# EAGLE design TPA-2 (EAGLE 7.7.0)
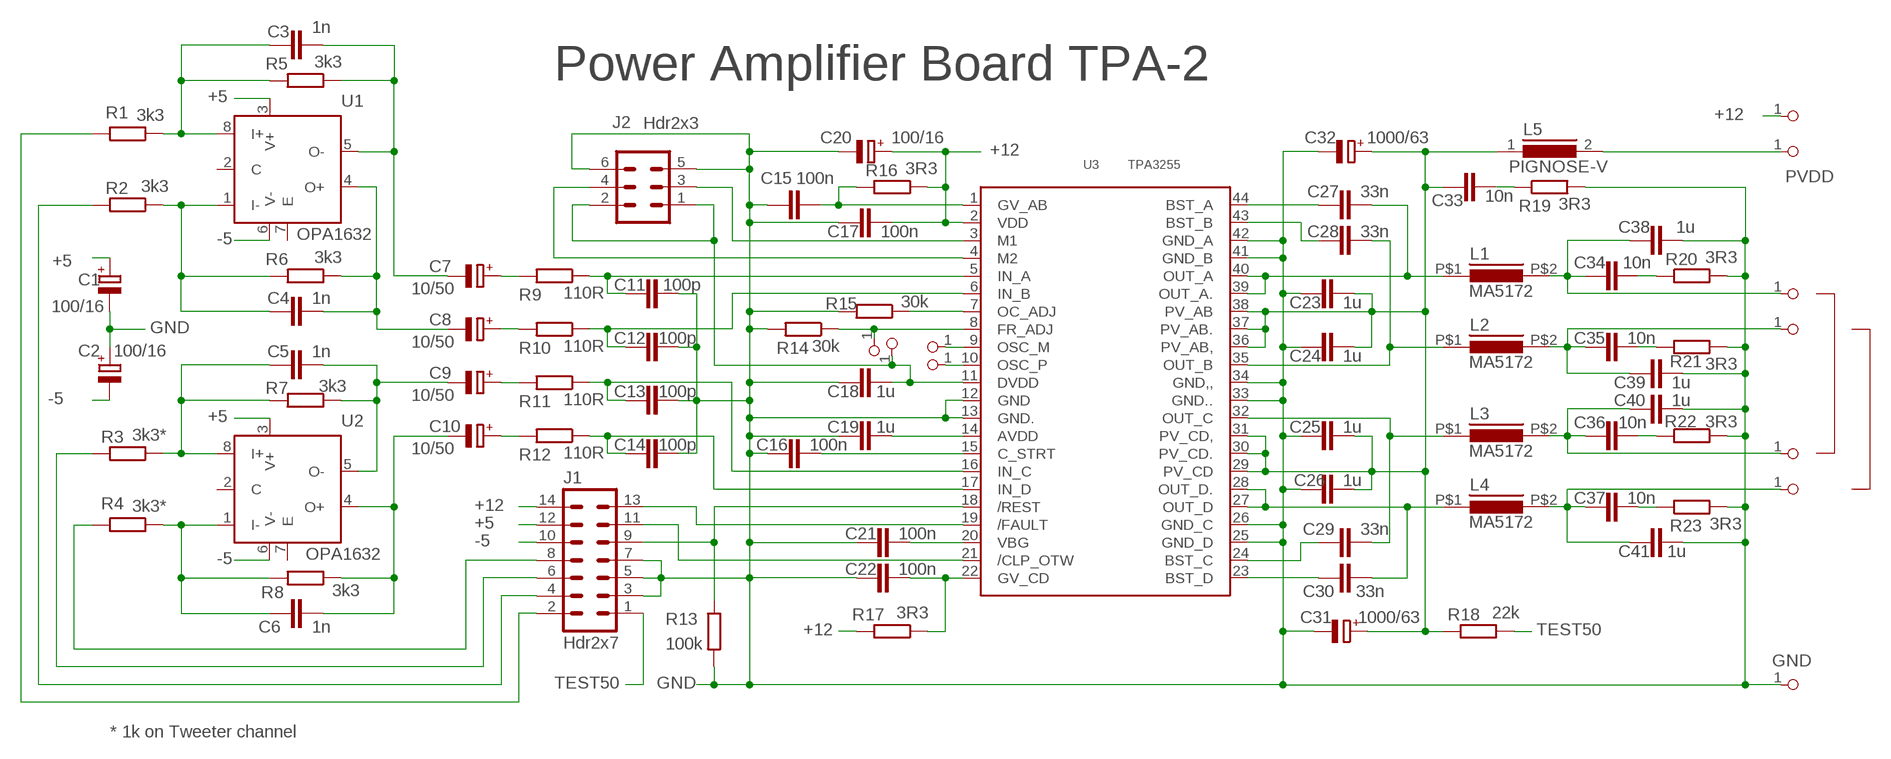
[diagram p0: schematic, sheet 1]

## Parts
12  PINHDR-1X1  [HDR1X1]
50  PINHDR-1X1  [HDR1X1]
A  PINHDR-1X1  [HDR1X1]
B  PINHDR-1X1  [HDR1X1]
C  PINHDR-1X1  [HDR1X1]
C1  100/16  CPOL-EUE2.5-6  [E2,5-6]
C2  100/16  CPOL-EUE2.5-6  [E2,5-6]
C3  1n  C-EUC0805  [C0805]
C4  1n  C-EUC0805  [C0805]
C5  1n  C-EUC0805  [C0805]
C6  1n  C-EUC0805  [C0805]
C7  10/50  CPOL-EUE2.5-6  [E2,5-6]
C8  10/50  CPOL-EUE2.5-6  [E2,5-6]
C9  10/50  CPOL-EUE2.5-6  [E2,5-6]
C10  10/50  CPOL-EUE2.5-6  [E2,5-6]
C11  100p  C-EUC0805  [C0805]
C12  100p  C-EUC0805  [C0805]
C13  100p  C-EUC0805  [C0805]
C14  100p  C-EUC0805  [C0805]
C15  100n  C-EUC1206  [C1206]
C16  100n  C-EUC1206  [C1206]
C17  100n  C-EUC1206  [C1206]
C18  1u  C-EUC1206  [C1206]
C19  1u  C-EUC1206  [C1206]
C20  100/16  CPOL-EUE2.5-6  [E2,5-6]
C21  100n  C-EUC1206  [C1206]
C22  100n  C-EUC1206  [C1206]
C23  1u  C-EUC1206  [C1206]
C24  1u  C-EUC1206  [C1206]
C25  1u  C-EUC1206  [C1206]
C26  1u  C-EUC1206  [C1206]
C27  33n  C-EUC1206  [C1206]
C28  33n  C-EUC1206  [C1206]
C29  33n  C-EUC1206  [C1206]
C30  33n  C-EUC1206  [C1206]
C31  1000/63  CPOL-EUE7.5-16  [E7,5-16]
C32  1000/63  CPOL-EUE7.5-16  [E7,5-16]
C33  10n  C-EUC1206  [C1206]
C34  10n  C-EUC1206  [C1206]
C35  10n  C-EUC1206  [C1206]
C36  10n  C-EUC1206  [C1206]
C37  10n  C-EUC1206  [C1206]
C38  1u  C-EU075-052X106  [C075-052X106]
C39  1u  C-EU075-052X106  [C075-052X106]
C40  1u  C-EU075-052X106  [C075-052X106]
C41  1u  C-EU075-052X106  [C075-052X106]
D  PINHDR-1X1  [HDR1X1]
DVDD  PINHDR-1X1  [HDR1X1]
FA  PINHDR-1X1  [HDR1X1]
G  PINHDR-1X1  [HDR1X1]
J1  Hdr2x7  PINHD-7X2  [MA07-2]
J2  Hdr2x3  PINHD-3X2  [MA03-2]
L1  MA5172  [L12X29]
L2  MA5172  [L12X29]
L3  MA5172  [L12X29]
L4  MA5172  [L12X29]
L5  PIGNOSE-V  INDUCTOR-PIGNOSE-V  [PIGNOSE]
OM  PINHDR-1X1  [HDR1X1]
OP  PINHDR-1X1  [HDR1X1]
R1  3k3  R-EU_0204/2V  [0204V]
R2  3k3  R-EU_0204/2V  [0204V]
R3  3k3*  R-EU_0204/2V  [0204V]
R4  3k3*  R-EU_0204/2V  [0204V]
R5  3k3  R-EU_0204/2V  [0204V]
R6  3k3  R-EU_0204/2V  [0204V]
R7  3k3  R-EU_0204/2V  [0204V]
R8  3k3  R-EU_0204/2V  [0204V]
R9  110R  R-EU_0204/2V  [0204V]
R10  110R  R-EU_0204/2V  [0204V]
R11  110R  R-EU_0204/2V  [0204V]
R12  110R  R-EU_0204/2V  [0204V]
R13  100k  R-EU_0204/2V  [0204V]
R14  30k  R-EU_0204/2V  [0204V]
R15  30k  R-EU_0204/2V  [0204V]
R16  3R3  R-EU_0204/2V  [0204V]
R17  3R3  R-EU_0204/2V  [0204V]
R18  22k  R-EU_0207/10  [0207/10]
R19  3R3  R-EU_0207/10  [0207/10]
R20  3R3  R-EU_0207/10  [0207/10]
R21  3R3  R-EU_0207/10  [0207/10]
R22  3R3  R-EU_0207/10  [0207/10]
R23  3R3  R-EU_0207/10  [0207/10]
U1  OPA1632  [SO08]
U2  OPA1632  [SO08]
U3  TPA3255  [HTSSOP-44]

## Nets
+5: C1.+ J1.12 U1.3(V+) U2.3(V+)
+12: 12.1 C17.2 C20.+ J1.14 R16.1 R17.2 U3.2(VDD)
-5: C2.- J1.10 U1.6(V-) U2.6(V-)
AVDD: C19.2 U3.14(AVDD)
BST_A: C27.1 U3.44(BST_A)
BST_B: C28.1 U3.43(BST_B)
BST_C: C29.1 U3.24(BST_C)
BST_D: C30.1 U3.23(BST_D)
CPLOTW: J1.11 U3.21(/CLP_OTW)
DVDD: C18.2 DVDD.1 J2.1 J2.2 U3.11(DVDD)
FLT: J1.13 U3.19(/FAULT)
FRADJ: FA.1 R14.1 U3.8(FR_ADJ)
GND: C1.- C2.+ C11.2 C12.2 C13.2 C14.2 C15.1 C16.1 C17.1 C18.1 C19.1 C20.- C21.1 C22.1 C23.1 C24.1 C25.1 C26.1 C31.- C32.- C38.1 C39.1 C40.1 C41.1 G.1 J1.3 J1.5 J1.7 J2.5 J2.6 R13.2 R14.2 R15.2 R19.2 R20.2 R21.2 R22.2 R23.2 U3.12(GND) U3.13(GND.) U3.25(GND_D) U3.26(GND_C) U3.33(GND..) U3.34(GND,,) U3.41(GND_B) U3.42(GND_A)
GVAB: C15.2 R16.2 U3.1(GV_AB)
GVCD: C22.2 R17.1 U3.22(GV_CD)
INA: C11.1 R9.1 U3.5(IN_A)
INB: C12.1 R10.1 U3.6(IN_B)
INC: C13.1 R11.1 U3.16(IN_C)
IND: C14.1 R12.1 U3.17(IN_D)
M1: J2.3 U3.3(M1)
M2: J2.4 U3.4(M2)
N$2: C37.1 R23.1
N$3: C37.2 C41.2 D.1 L4.P$2
N$4: A.1 C34.2 C38.2 L1.P$2
N$5: C36.2 C40.2 C.1 L3.P$2
N$9: B.1 C35.2 C39.2 L2.P$2
N$18: C7.+ R9.2
N$20: C34.1 R20.1
N$23: C35.1 R21.1
N$26: C3.1 R1.1 R5.2 U1.8(I+)
N$27: C36.1 R22.1
N$28: C33.1 R19.1
N$30: C8.+ R10.2
N$35: J1.8 R4.2
N$36: J1.6 R3.2
N$37: J1.4 R2.2
N$40: J1.2 R1.2
N$41: 50.1 L5.2
N$42: C9.+ R11.2
N$43: C10.+ R12.2
N$45: C4.1 R2.1 R6.2 U1.1(I-)
N$50: C4.2 C8.- R6.1 U1.4(O+)
N$51: C3.2 C7.- R5.1 U1.5(O-)
N$52: C5.2 C9.- R7.1 U2.5(O-)
N$53: C5.1 R3.1 R7.2 U2.8(I+)
N$55: C6.1 R4.1 R8.2 U2.1(I-)
N$56: C6.2 C10.- R8.1 U2.4(O+)
OM: OM.1 U3.9(OSC_M)
OP: OP.1 U3.10(OSC_P)
OSCADJ: R15.1 U3.7(OC_ADJ)
OUT_A: C27.2 L1.P$1 U3.39(OUT_A.) U3.40(OUT_A)
OUT_B: C28.2 L2.P$1 U3.35(OUT_B)
OUT_C: C29.2 L3.P$1 U3.32(OUT_C)
OUT_D: C30.2 L4.P$1 U3.27(OUT_D) U3.28(OUT_D.)
PVDD: C23.2 C24.2 C25.2 C26.2 C31.+ C32.+ C33.2 L5.1 R18.1 U3.29(PV_CD) U3.30(PV_CD.) U3.31(PV_CD,) U3.36(PV_AB,) U3.37(PV_AB.) U3.38(PV_AB)
RST: J1.9 R13.1 U3.18(/REST)
STRT: C16.2 U3.15(C_STRT)
TEST50: J1.1 R18.2
VBG: C21.2 U3.20(VBG)
Unconnected: U1.2(C) U1.7(E) U2.2(C) U2.7(E)

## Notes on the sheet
- Power Amplifier Board TPA-2
- * 1k on Tweeter channel

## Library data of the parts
12 50 A B C D DVDD FA G OM OP = Header:PINHDR-1X1
C1 C2 C7-C10 C20 C31 C32 = Passive:CPOL-EU: POLARIZED CAPACITOR, European symbol
C3-C6 C11-C19 C21-C30 C33-C41 = Passive:C-EU: CAPACITOR, European symbol
J1 = Header:PINHD-7X2: PIN HEADER
J2 = Header:PINHD-3X2: PIN HEADER
L1-L4 = Passive:MA5172
L5 = Passive:INDUCTOR: INDUCTOR
R1-R23 = AJANLIB:R-EU_: RESISTOR, European symbol
U1 U2 = IC_Lin:OPA1632
U3 = MotorDrive:TPA3255: 4-2-1 Channel Class D Audio Power stage

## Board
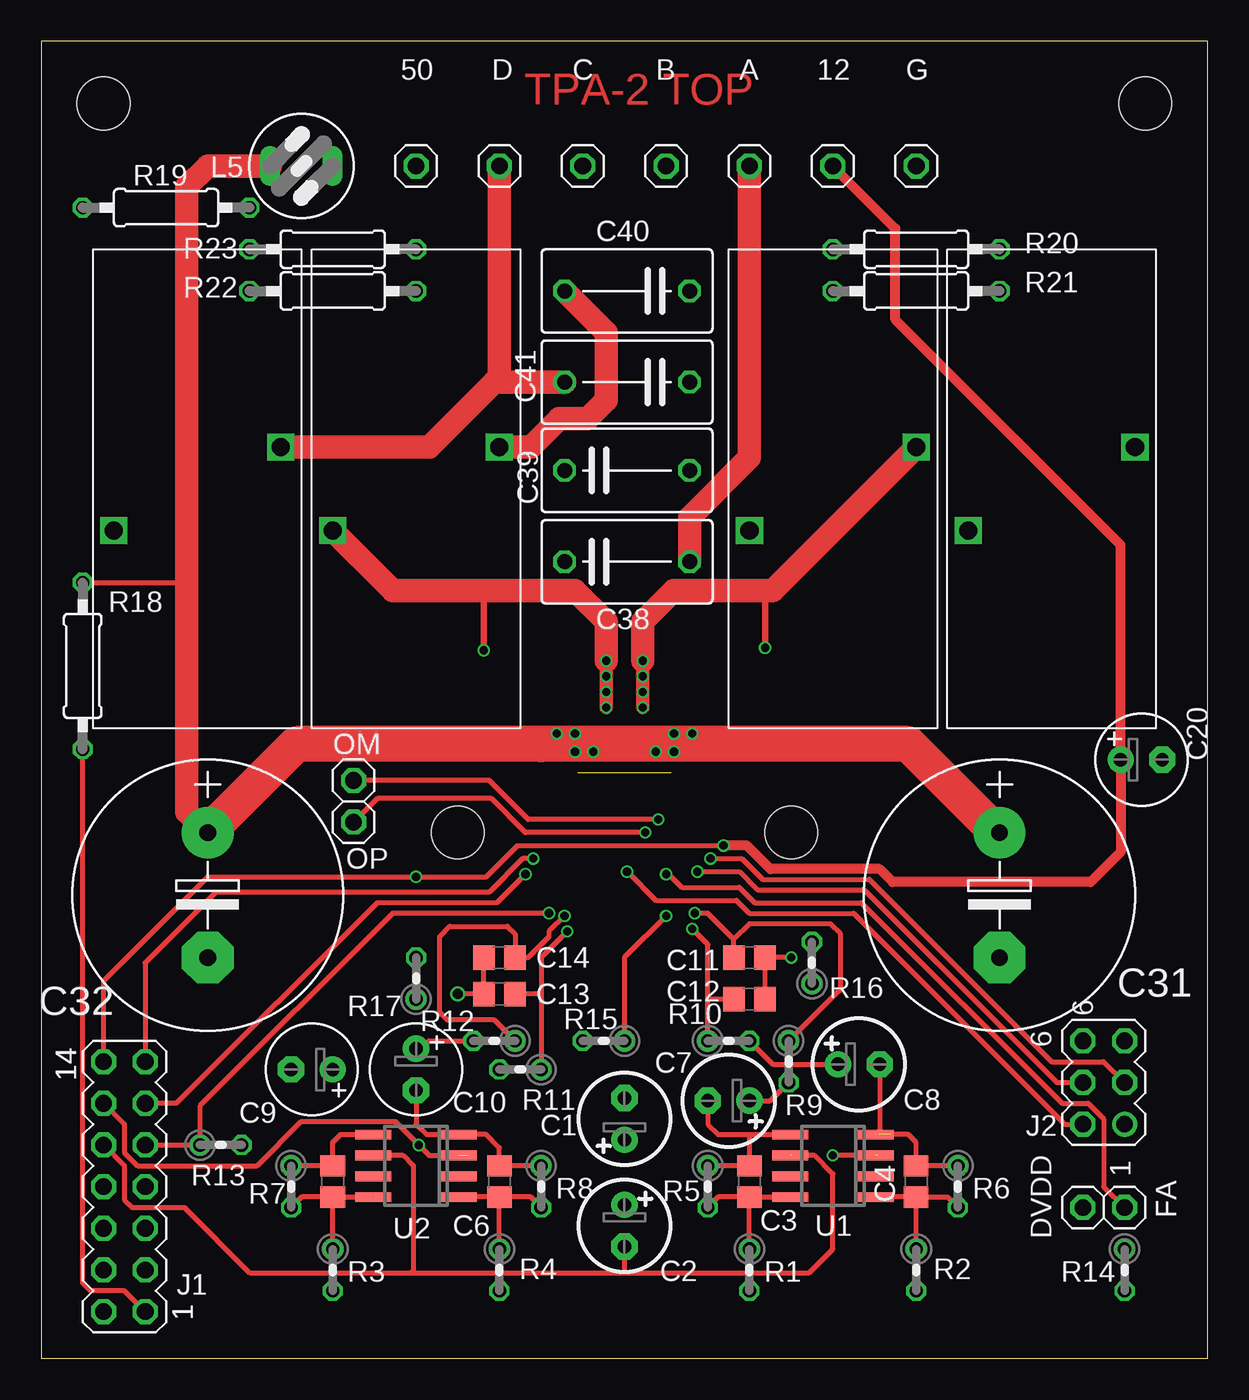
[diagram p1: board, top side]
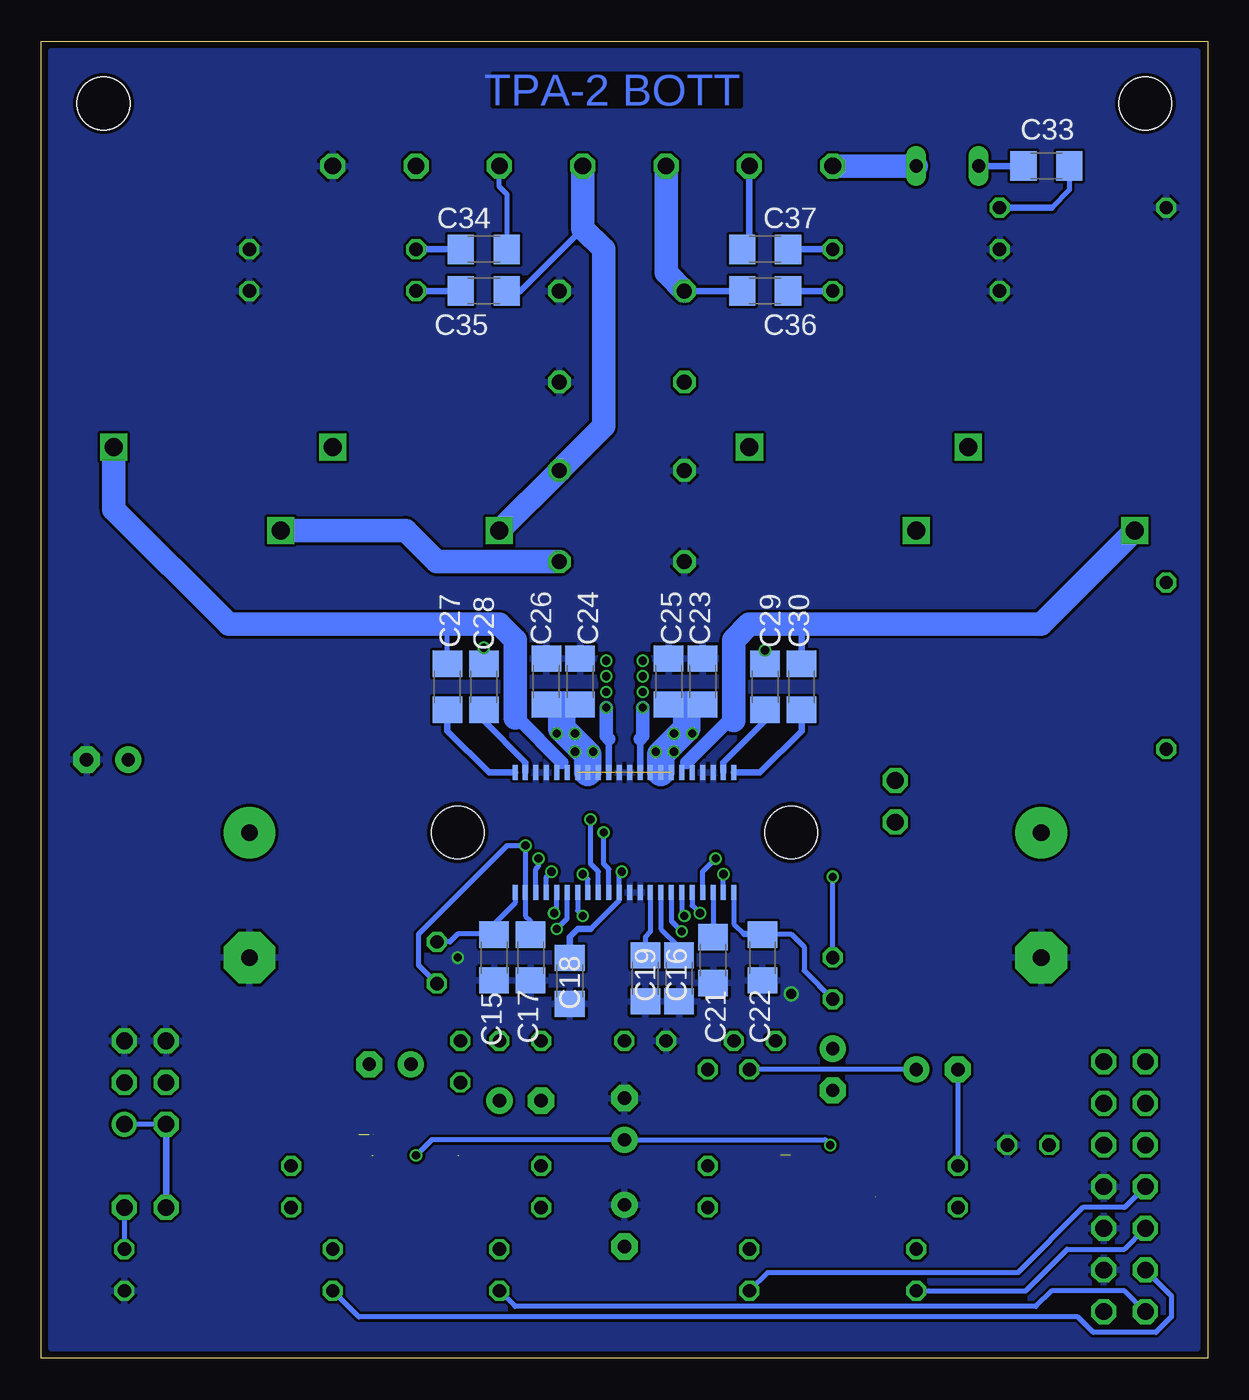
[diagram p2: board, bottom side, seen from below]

Size 71.12 x 80.33 mm. Coordinates in mm from the lower left corner, seen from the top.
Outline: 0,0 71.12,0 71.12,80.33 0,80.31 0,0
Copper layers (1*16): Top 0.035mm / dielectric 1.55mm / Bottom 0.035mm
Design rules "eC_2Layer_PClass6_BaseCopperO35 *": minimum track width 0.15mm, minimum drill 0.35mm, track to track 0.175mm, track to pad 0.175mm, pad to pad 0.175mm, via to via 0.175mm, smd to smd 0mil, copper to edge 0.25mm, drill to drill 0.35mm, minimum pad ring 0.175mm, minimum via ring 0.125mm, stop-mask expansion 0mil, vias tented up to drill 0.45mm, thermal gap 0.2mm
Holes 3.2 mm at 45.72,32.07 25.4,32.07 67.31,76.52 3.81,76.52

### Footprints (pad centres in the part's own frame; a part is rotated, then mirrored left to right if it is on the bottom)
HDR1X1 = drill 1.016 octagon: 1 0,0
E2,5-6 = drill 0.813 pad 1.6: + -1.27,0 | drill 0.813 pad 1.6 octagon: - 1.27,0
C0805 = smd 1.3 x 1.5: 1 -0.95,0; 2 0.95,0
C1206 = smd 1.6 x 1.8: 1 -1.4,0; 2 1.4,0
E7,5-16 = drill 1.016 pad 3.15: + -3.81,0 | drill 1.016 pad 3.15 octagon: - 3.81,0
C075-052X106 = drill 0.914 octagon: 1 -3.81,0; 2 3.81,0
MA07-2 = drill 1.016 octagon: 1 -7.62,-1.27; 2 -7.62,1.27; 3 -5.08,-1.27; 4 -5.08,1.27; 5 -2.54,-1.27; 6 -2.54,1.27; 7 0,-1.27; 8 0,1.27; 9 2.54,-1.27; 10 2.54,1.27; 11 5.08,-1.27; 12 5.08,1.27; 13 7.62,-1.27; 14 7.62,1.27
MA03-2 = drill 1.016: 1 -2.54,-1.27 | drill 1.016 octagon: 2 -2.54,1.27; 3 0,-1.27; 4 0,1.27; 5 2.54,-1.27; 6 2.54,1.27
L12X29 = drill 1.1 square: P$1 -5.08,-2.54; P$2 5.08,2.54
PIGNOSE = drill 0.813 long: 1 0,1.905; 2 0,-1.905
0204V = drill 0.813 octagon: 1 -1.27,0; 2 1.27,0
0207/10 = drill 0.813 octagon: 1 -5.08,0; 2 5.08,0
SO08 = smd 0.6 x 2.2: 1 -1.905,-2.6; 2 -0.635,-2.6; 3 0.635,-2.6; 4 1.905,-2.6; 5 1.905,2.6; 6 0.635,2.6; 7 -0.635,2.6; 8 -1.905,2.6
HTSSOP-44 = smd 0.914 x 0.305: 1 -3.651,6.35; 2 -3.651,5.715; 3 -3.651,5.08; 4 -3.651,4.445; 5 -3.651,3.81; 6 -3.651,3.175; 7 -3.651,2.54; 8 -3.651,1.905; 9 -3.651,1.27; 10 -3.651,0.635; 11 -3.651,0; 12 -3.651,-0.635; 13 -3.651,-1.27; 14 -3.651,-1.905; 15 -3.651,-2.54; 16 -3.651,-3.175; 17 -3.651,-3.81; 18 -3.651,-4.445; 19 -3.651,-5.08; 20 -3.651,-5.715; 21 -3.651,-6.35; 22 -3.651,-6.985; 23 3.651,-6.985; 24 3.651,-6.35; 25 3.651,-5.715; 26 3.651,-5.08; 27 3.651,-4.445; 28 3.651,-3.81; 29 3.651,-3.175; 30 3.651,-2.54; 31 3.651,-1.905; 32 3.651,-1.27; 33 3.651,-0.635; 34 3.651,0; 35 3.651,0.635; 36 3.651,1.27; 37 3.651,1.905; 38 3.651,2.54; 39 3.651,3.175; 40 3.651,3.81; 41 3.651,4.445; 42 3.651,5.08; 43 3.651,5.715; 44 3.651,6.35

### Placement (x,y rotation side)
12  48.26,72.71 90 top
50  22.86,72.71 90 top
A  43.18,72.71 90 top
B  38.1,72.71 90 top
C  33.02,72.71 90 top
C1  35.56,14.61 90 top
C2  35.56,8.1 270 top
C3  43.18,10.79 90 top
C4  53.34,10.79 90 top
C5  17.78,10.79 90 top
C6  27.94,10.79 90 top
C7  41.91,15.72 180 top
C8  49.85,17.94 0 top
C9  16.51,17.62 180 top
C10  22.86,17.62 270 top
C11  43.18,24.45 0 top
C12  43.18,21.91 0 top
C13  27.94,22.23 180 top
C14  27.94,24.45 180 top
C15  43.5,24.45 90 bottom
C16  32.23,23.18 90 bottom
C17  41.27,24.45 90 bottom
C18  38.89,23.02 90 bottom
C19  34.29,23.18 90 bottom
C20  67.07,36.51 0 top
C21  30.16,24.29 90 bottom
C22  27.15,24.45 90 bottom
C23  30.8,41.27 270 bottom
C24  38.26,41.27 270 bottom
C25  32.86,41.27 270 bottom
C26  40.32,41.27 270 bottom
C27  46.35,40.96 90 bottom
C28  44.13,40.96 90 bottom
C29  26.99,40.96 90 bottom
C30  24.77,40.96 90 bottom
C31  58.42,28.26 270 top
C32  10.16,28.26 270 top
C33  9.84,72.71 180 bottom
C34  44.13,67.63 0 bottom
C35  44.13,65.09 0 bottom
C36  26.99,65.09 180 bottom
C37  26.99,67.63 180 bottom
C38  35.72,48.58 0 top
C39  35.72,54.15 0 top
C40  35.72,65.09 180 top
C41  35.72,59.53 180 top
D  27.94,72.71 90 top
DVDD  63.5,9.21 90 top
FA  66.04,9.21 90 top
G  53.34,72.71 90 top
J1  5.08,10.48 90 top
J2  64.77,16.83 90 top
L1  61.59,53.02 180 top
L2  48.26,53.02 180 top
L3  22.86,53.02 0 top
L4  9.53,53.02 0 top
L5  15.88,72.71 90 top
OM  19.05,35.24 90 top
OP  19.05,32.7 90 top
R1  43.18,5.4 270 top
R2  53.34,5.4 270 top
R3  17.78,5.4 270 top
R4  27.94,5.4 270 top
R5  40.64,10.48 270 top
R6  55.88,10.48 270 top
R7  15.24,10.48 270 top
R8  30.48,10.48 270 top
R9  45.56,18.1 270 top
R10  41.91,19.37 0 top
R11  29.21,17.62 180 top
R12  27.62,19.37 180 top
R13  10.95,13.02 0 top
R14  66.04,5.4 270 top
R15  34.29,19.37 180 top
R16  46.99,24.13 90 top
R17  22.86,23.18 90 top
R18  2.54,42.23 270 top
R19  7.62,70.17 180 top
R20  53.34,67.63 0 top
R21  53.34,65.09 0 top
R22  17.78,65.09 180 top
R23  17.78,67.63 180 top
U1  48.26,11.75 90 top
U2  22.86,11.75 90 top
U3  35.88,32.07 90 bottom

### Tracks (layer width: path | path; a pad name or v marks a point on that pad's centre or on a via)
+5  (via drill 0.5)  (2 unrouted)
  Top 0.305: J1.12 5.08,14.29 5.08,12.54 5.87,11.75 13.18,11.75 15.88,14.45 21.59,14.45 v23.02,13.02 23.65,12.38 26.04,12.38 | 50.96,12.38 v48.26,12.38
  Bottom 0.305: v23.02,13.02 23.34,13.34 C1.+ 47.31,13.34 v48.26,12.38
+12  (via drill 0.5)
  Top 0.305: v41.59,31.27 29.05,31.27 27.15,29.37 v22.86,29.37 10.16,29.37 3.81,23.02 J1.14
  Top 0.61: 12.1 52.07,68.9 52.07,63.34 65.8,49.61 C20.+ 65.8,30.88 63.98,29.05 51.91,29.05 51.12,29.84 44.45,29.84 43.02,31.27 v41.59,31.27
  Bottom 0.305: C17.2 41.27,26.67 41.59,26.99 U3.2 v41.59,31.27 42.7,31.27 48.1,25.88 48.1,23.97 R16.1 | R17.2 v22.86,29.37
-5  (1 unrouted)
  Top 0.305: J1.10 5.08,11.75 5.08,9.68 5.56,9.21 8.73,9.21 12.7,5.24 22.54,5.24 | 22.54,5.24 22.7,5.4 22.7,11.75 22.07,12.38 U2.6 | 22.54,5.24 35.56,5.24 | 35.56,5.24 46.83,5.24 48.26,6.67 48.26,11.27 47.15,12.38 45.72,12.38 | C2.- 35.56,5.24
AVDD
  Bottom 0.305: U3.14 33.97,26.04 34.29,25.72 C19.2
BST_A
  Bottom 0.406: C27.1 46.35,38.26 43.81,35.72 U3.44
BST_B
  Bottom 0.406: C28.1 44.13,38.89 41.59,36.35 U3.43
BST_C
  Bottom 0.406: C29.1 26.99,38.89 29.53,36.35 U3.24
BST_D
  Bottom 0.406: C30.1 24.77,38.26 27.3,35.72 U3.23
CPLOTW  (via drill 0.5)
  Top 0.305: v29.53,29.53 27.78,27.78 20.48,27.78 8.26,15.56 J1.11
  Bottom 0.305: U3.21 v29.53,29.53
DVDD  (via drill 0.5)
  Top 0.305: v35.72,29.69 37.47,27.94 42.39,27.94 43.18,27.15 49.53,27.15 62.39,14.29 J2.2
  Bottom 0.305: 38.89,25.24 38.89,24.92 | v35.72,29.69 35.88,29.53 U3.11 35.88,27.94 37.62,26.19 | J2.2 J2.1
  Bottom 0.406: J2.2 DVDD.1 | 37.62,26.19 38.42,26.19 38.89,25.72 38.89,25.24 | 38.89,24.92 C18.2
FLT  (via drill 0.5)
  Top 0.305: v30,30.48 29.37,30.48 27.3,28.42 10.64,28.42 6.35,24.13 J1.13
  Bottom 0.305: U3.19 30.8,29.69 v30,30.48
FRADJ  (via drill 0.5)
  Top 0.305: v38.1,29.53 38.26,29.53 39.05,28.73 42.55,28.73 43.5,27.78 50.01,27.78 62.23,15.56 63.82,15.56 64.77,14.61 64.77,10.48 FA.1
  Bottom 0.305: U3.8 37.78,29.21 v38.1,29.53 | FA.1 R14.1
GND  (via drill 0.5, 0.6)
  Top 0.305: C12.2 C11.2 v45.72,24.45 | C14.2 C13.2 v25.4,22.23
  pour Bottom: 0.64,79.69 70.48,79.69 70.48,0.64 0.64,0.64
GVAB
  Bottom 0.305: U3.1 42.23,27.78 43.5,26.51 C15.2 43.95,25.85 43.97,25.88 45.72,25.88 46.2,25.4 R16.2
GVCD
  Bottom 0.305: U3.22 28.89,26.51 28.26,25.88 25.4,25.88 24.61,25.08 24.61,23.65 R17.1
  Bottom 0.406: 28.26,25.88 27.18,25.88 C22.2
INA  (via drill 0.5)
  Top 0.305: 42.23,25.56 C11.1 42.23,23.97 | 42.23,25.56 40.64,27.15 v39.85,27.15 | R9.1 48.74,22.54 48.74,25.88 48.1,26.51 43.19,26.51 42.23,25.56
  Bottom 0.305: v39.85,27.15 39.69,27.3 U3.5
INB  (via drill 0.5)
  Top 0.305: v39.69,26.19 40.64,25.24 40.64,21.91 | R10.1 40.64,21.91 | C12.1 40.64,21.91
  Bottom 0.305: v39.69,26.19 39.05,26.83 U3.6
INC  (via drill 0.5)
  Top 0.305: v32.07,26.04 30.48,24.45 30.48,22.23 | 30.48,22.23 R11.1 | 30.48,22.23 C13.1
  Bottom 0.305: U3.16 32.7,26.67 v32.07,26.04
IND  (via drill 0.5)
  Top 0.305: v31.91,26.99 30.96,26.04 30.96,25.72 29.69,24.45 C14.1 | R12.1 27.62,20.64 24.77,20.64 24.29,21.11 24.29,25.72 24.92,26.35 28.42,26.35 28.89,25.88 C14.1 | C14.1
  Bottom 0.305: U3.17 32.07,27.15 v31.91,26.99
M1  (via drill 0.5)
  Top 0.305: v40.8,30.48 42.7,30.48 43.97,29.21 50.48,29.21 61.59,18.1 64.77,18.1 J2.3
  Bottom 0.305: U3.3 40.96,29.84 40.8,30 v40.8,30.48
M2  (via drill 0.5)
  Top 0.305: v40.01,29.69 42.55,29.69 43.66,28.57 50.16,28.57 61.91,16.83 J2.4
  Bottom 0.305: U3.4 40.32,29.37 v40.01,29.69
N$2
  Bottom 0.406: C37.1 R23.1
N$3
  Top 1.422: L4.P$2 23.65,55.56 27.62,59.53 27.94,59.53 | C41.2 27.94,59.53 | 27.94,59.53 D.1
  Bottom 0.305: 27.94,68.08 C37.2
  Bottom 0.406: D.1 27.94,68.08
N$4
  Top 1.422: A.1 43.18,54.93 39.53,51.28 C38.2
  Bottom 0.305: C34.2 42.7,67.63 42.7,70.96 43.18,71.44 A.1
  Bottom 1.422: L1.P$2 48.9,50.48 46.99,48.58 C38.2
N$5
  Top 1.422: C40.2 34.45,62.55 34.45,58.42 33.34,57.31 31.59,57.31 29.84,55.56 L3.P$2
  Bottom 0.406: C40.2 C36.2
  Bottom 1.422: C.1 33.02,66.2 C40.2
N$9
  Bottom 0.406: C35.2 41.91,65.09 38.1,68.9
  Bottom 1.422: 43.18,50.5 L2.P$2 39.51,54.15 C39.2 36.83,56.85 36.83,67.63 38.1,68.9 B.1
N$18
  Top 0.305: C7.+ 44.45,15.72 R9.2
N$20
  Bottom 0.406: C34.1 R20.1
N$23
  Bottom 0.406: C35.1 R21.1
N$26
  Top 0.305: C3.1 | C3.1 41.28,9.85 R5.2 | R1.1 C3.1 | C3.1 U1.8
N$27
  Bottom 0.406: C36.1 R22.1
N$28
  Bottom 0.305: C33.1 8.44,71.25 9.53,70.17
  Bottom 0.406: 9.53,70.17 R19.1
N$30
  Top 0.305: R10.2 44.61,17.94 C8.+
N$35
  Bottom 0.305: J1.8 5.08,9.21 7.62,9.21 11.59,5.24 26.83,5.24 R4.2
N$36
  Bottom 0.305: R3.2 11.11,4.13 8.57,6.67 5.08,6.67 J1.6
N$37
  Bottom 0.305: J1.4 2.22,3.81 2.22,2.54 3.17,1.59 6.99,1.59 7.94,2.54 51.75,2.54 R2.2
N$40
  Bottom 0.305: J1.2 5.08,4.13 9.53,4.13 10.48,3.17 42.23,3.17 R1.2
N$41
  Bottom 1.422: 50.1 L5.2
N$42
  Bottom 0.305: C9.+ R11.2
N$43
  Top 0.305: R12.2 23.65,19.37 23.18,18.89 C10.+
N$44  (via drill 0.5)
  other vias: 32.54,36.99
N$45
  Top 0.305: C4.1 | C4.1 55.24,9.85 R6.2 | R2.1 C4.1 | C4.1 53.34,10.16 | C4.1 U1.1
N$50  (2 unrouted)
  Top 0.305: R6.1 C4.2 53.34,13.18 52.86,13.65 51.75,13.65 | C8.- 51.12,13.66 U1.4
N$51
  Top 0.305: 43.18,13.65 C3.2 R5.1 | 43.18,13.65 41.27,13.65 40.64,14.29 C7.- | 43.18,13.65 U1.5
N$52
  Top 0.305: C5.2 | C5.2 17.78,13.18 18.26,13.65 U2.5 | C5.2 R7.1
  Bottom 0.305: C9.- R7.1
N$53  (1 unrouted)
  Top 0.305: R3.1 C5.1 | C5.1 15.88,9.85 R7.2 | C5.1 U2.8
N$55
  Top 0.305: R4.1 27.94,9.21 | 27.94,9.21 C6.1 29.84,9.84 R8.2 | 27.94,9.21 27.3,9.84 U2.1
N$56
  Top 0.305: R8.1 C6.2 27.94,12.86 27.15,13.65 U2.4 23.5,13.65 22.86,14.29 C10.-
N$57  (via drill 0.5)
  other vias: 33.66,36.99
N$58  (via drill 0.5)
  other vias: 37.47,36.99
N$59  (via drill 0.5)
  other vias: 38.58,36.99
N$60  (via drill 0.5)
  other vias: 38.58,38.1
N$61  (via drill 0.5)
  other vias: 39.69,38.1
N$62  (via drill 0.5)
  other vias: 32.54,38.1
OM  (via drill 0.5)
  Top 0.305: v37.62,32.86 29.69,32.86 27.3,35.24 OM.1
  Bottom 0.305: U3.9 37.15,29.69 37.62,30.16 v37.62,32.86
OP  (via drill 0.5)
  Top 0.305: v36.83,32.07 29.53,32.07 27.46,34.13 20.48,34.13 OP.1
  Bottom 0.305: U3.10 36.51,29.84 36.83,30.16 v36.83,32.07
OSCADJ  (via drill 0.5)
  Top 0.305: v38.1,26.99 35.56,24.45 R15.1
  Bottom 0.305: U3.7 38.42,27.3 v38.1,26.99
OUT_A
  Bottom 0.254: U3.40 39.69,36.04 39.37,36.35 39.05,36.04 U3.39
  Bottom 0.305: C27.2 46.35,44.77
  Bottom 0.813: 42.23,39.05 42.07,39.05 39.37,36.35
  Bottom 1.422: 42.23,39.05 42.23,43.81 43.18,44.77 46.35,44.77 59.69,44.77 66.67,51.75 L1.P$1
OUT_B  (via drill 0.5)
  Top 0.406: v44.13,43.34 44.13,46.83
  Top 0.813: v36.67,42.55 v36.67,41.59 v36.67,40.64 v36.67,39.69
  Top 1.422: v36.67,42.55 36.67,44.93 38.58,46.83 44.13,46.83 44.61,46.83 L2.P$1
  Bottom 0.406: 36.51,37.78 U3.35 | C28.2 v44.13,43.34
  Bottom 0.813: v36.67,39.69 36.67,37.94 36.51,37.78
OUT_C  (via drill 0.5)
  Top 0.406: v26.99,43.18 26.99,46.83
  Top 0.813: v34.45,42.55 v34.45,41.59 v34.45,40.64 v34.45,39.69
  Top 1.422: v34.45,42.55 34.45,44.93 32.54,46.83 26.99,46.83 21.43,46.83 L3.P$1
  Bottom 0.406: U3.32 34.61,37.78 | C29.2 v26.99,43.18
  Bottom 0.813: v34.45,39.69 34.45,37.94 34.61,37.78
OUT_D
  Bottom 0.254: U3.28 32.07,36.04 31.75,36.35 | U3.27 31.43,36.35 31.59,36.51
  Bottom 0.305: 28.89,38.89 29.21,38.89
  Bottom 0.406: 24.77,44.77 C30.2
  Bottom 0.813: 29.21,38.89 31.59,36.51 31.75,36.35
  Bottom 1.422: 28.89,38.89 28.89,43.81 27.94,44.77 24.77,44.77 10.16,44.77 L4.P$1
PVDD  (via drill 0.5)  (5 unrouted)
  Top 0.305: R18.1 8.89,47.31
  Top 0.406: v31.43,38.1 30.48,37.47
  Top 1.016: C31.+ 58.26,32.07
  Top 1.422: L5.1 10.16,72.71 8.89,71.44 8.89,47.31 8.89,33.34 C32.+
  Top 2.184: 58.26,32.07 52.86,37.47 30.48,37.47 15.56,37.47 C32.+
  Bottom 0.305: 38.26,39.85 C24.2
  Bottom 0.406: 39.37,39.69 40.16,39.69 40.32,39.85 C26.2 | C25.2 32.86,39.85 31.75,39.85 30.8,39.85 C23.2 31.27,40.01 31.91,39.37 31.59,39.21 v31.43,38.1 32.7,36.99 32.86,37.15 33.34,37.15 33.34,36.83 | L5.1 C33.2 | 39.21,39.85 38.29,39.85 C24.2 | 38.26,39.85
  Bottom 1.676: U3.30 33.34,36.83 31.75,38.42 31.75,39.85 | U3.37 37.78,36.83 39.37,38.42 39.37,39.69 39.21,39.85
RST  (via drill 0.5)
  Top 0.305: v30.96,27.15 21.43,27.15 9.68,15.4 R13.1 J1.9
  Bottom 0.305: U3.18 31.43,27.62 v30.96,27.15
STRT
  Bottom 0.305: U3.15 33.34,26.19 32.23,25.08 C16.2
TEST50
  Top 0.305: J1.1 5.08,4.13 3.02,4.13 2.54,4.6 R18.2
VBG
  Bottom 0.305: U3.20 C21.2

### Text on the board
Top: TPA-2 TOP
Bottom: TPA-2 BOTT
tNames: 6 | 14 | 1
